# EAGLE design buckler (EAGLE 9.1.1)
AUTHOR: Branden Ghena; REV: C; TITLE: Berkeley Buckler

## Sheet 1 of 3: Headers
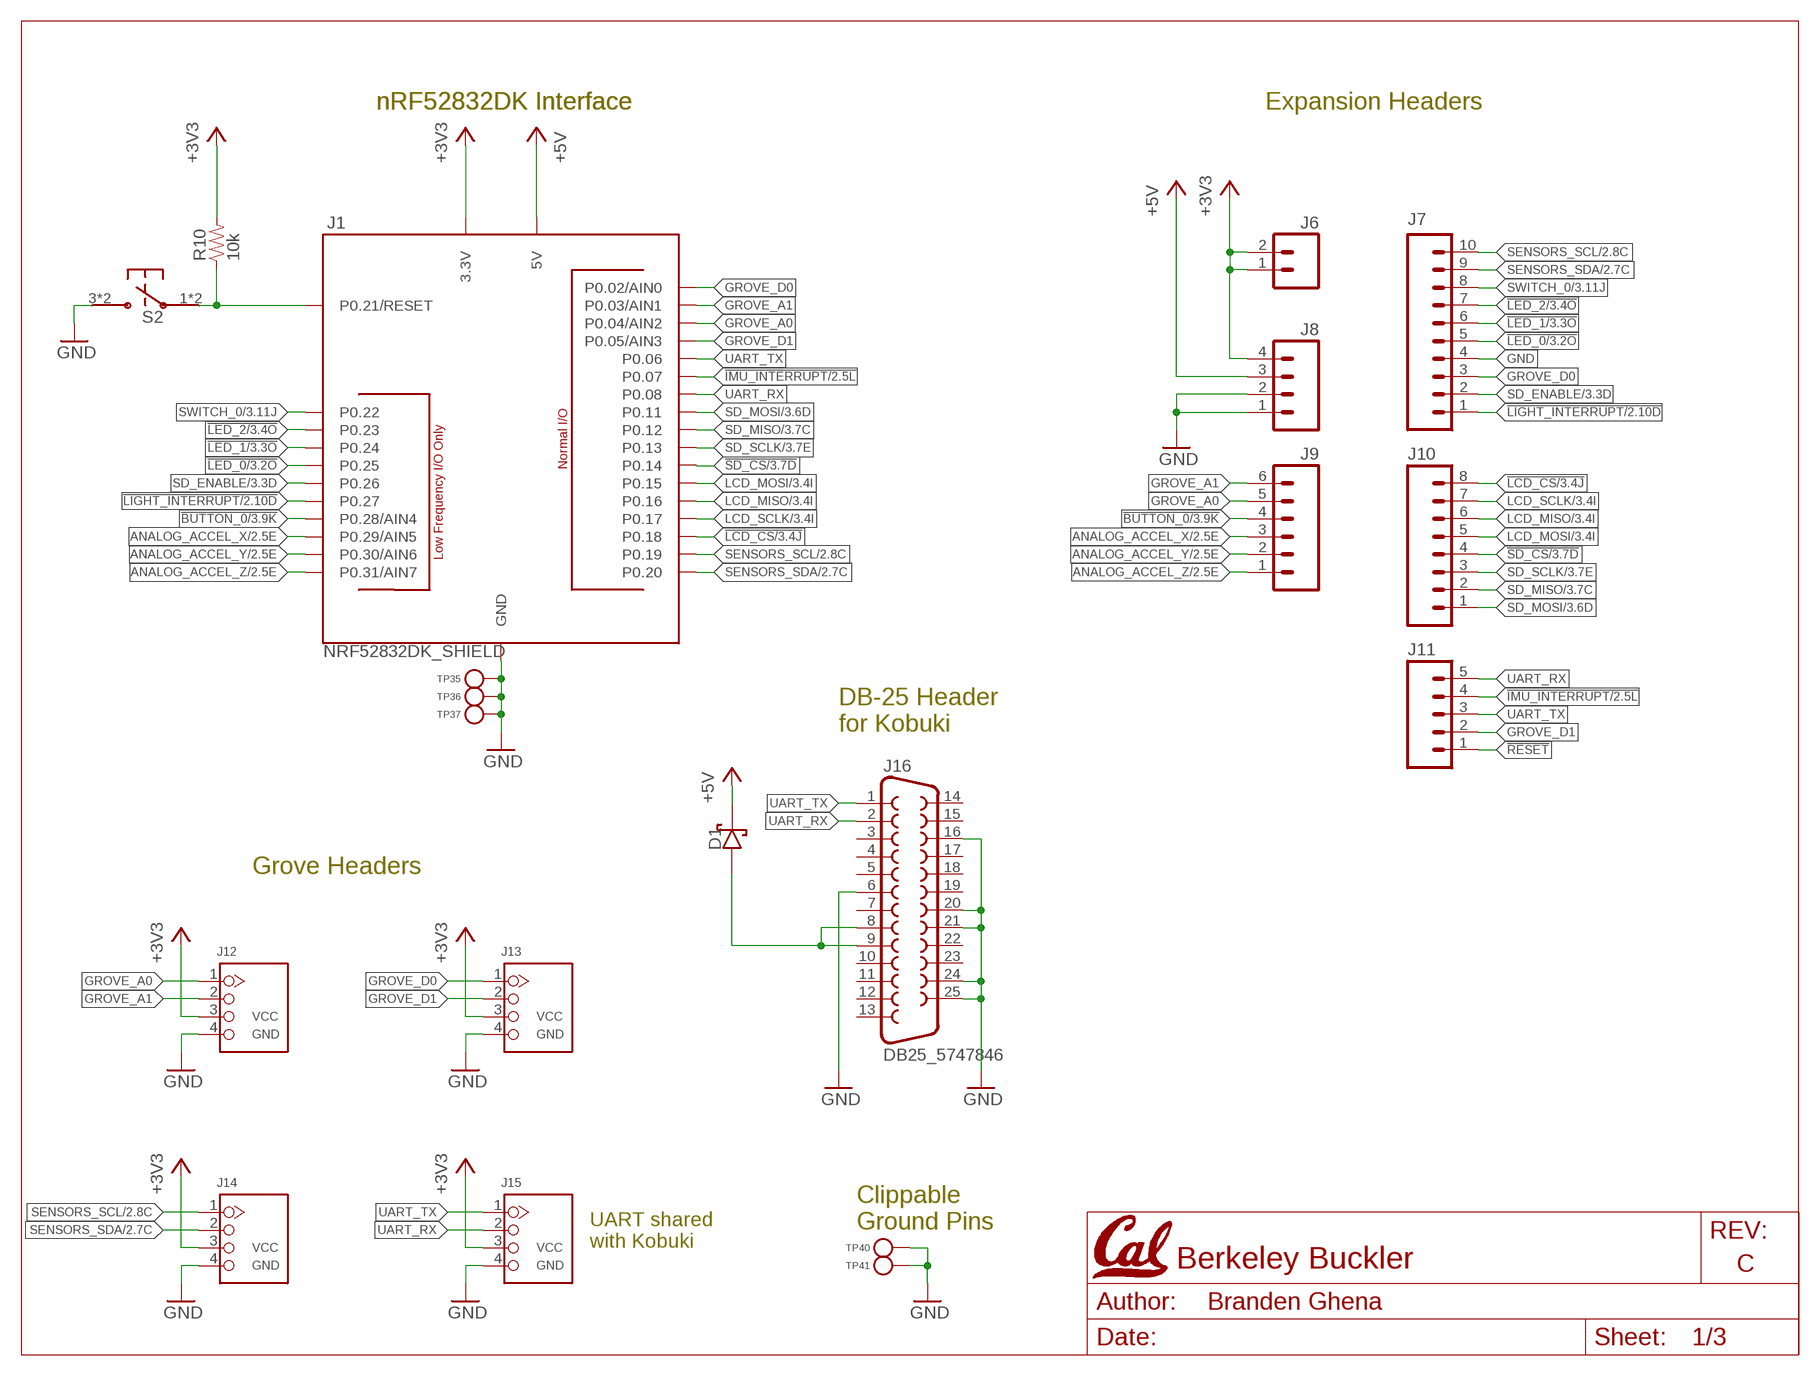
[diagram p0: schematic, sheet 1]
U$1 (LETTER_L_CAL): HEIGHT: 8.5in; WIDTH: 11in

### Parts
D1  DIODE_SCHOTTKYSOD323  [SOD323]
J1  NRF52832DK_SHIELD  [NRF52832DK_SHIELD]
J6  M02PTH  [1X02]
J7  M10"  [1X10]
J8  M04PTH  [1X04]
J9  M06SIP  [1X06]
J10  M081X08  [1X08]
J11  M05PTH  [1X05]
J12  GROVE-CONNECTOR-DIP(4P-2.0)  [HW4-2.0]
J13  GROVE-CONNECTOR-DIP(4P-2.0)  [HW4-2.0]
J14  GROVE-CONNECTOR-DIP(4P-2.0)  [HW4-2.0]
J15  GROVE-CONNECTOR-DIP(4P-2.0)  [HW4-2.0]
J16  DB25_5747846  [DB25_5747846]
R10  10k  RESISTOR0402_RES  [0402_RES]
S2  PTS645SM43SMTR92  [PTS645]
TP35  TEST_POINT_0.040IN  [TESTPOINT_0.040IN]
TP36  TEST_POINT_0.040IN  [TESTPOINT_0.040IN]
TP37  TEST_POINT_0.040IN  [TESTPOINT_0.040IN]
TP40  TEST_POINT_0.078IN  [TESTPOINT_0.078IN]
TP41  TEST_POINT_0.078IN  [TESTPOINT_0.078IN]

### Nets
5V_IN: D1.P$2(ANODE) J16.8 J16.9
!BUTTON_0: J1.P0.28(P0.28/AIN4) J9.4 ; also sheet 3
!IMU_INTERRUPT: J1.P0.07 J11.4 ; also sheet 2
!LCD_CS: J1.P0.18 J10.8 ; also sheet 3
!LED_0: J1.P0.25 J7.5 ; also sheet 3
!LED_1: J1.P0.24 J7.6 ; also sheet 3
!LED_2: J1.P0.23 J7.7 ; also sheet 3
!LIGHT_INTERRUPT: J1.P0.27 J7.1 ; also sheet 2
!RESET: J1.P0.21(P0.21/RESET) J11.1 R10.1 S2.1 S2.2
!SD_CS: J1.P0.14 J10.4 ; also sheet 3
+3V3: J1.3.3V@0(3.3V) J1.3.3V@1(3.3V) J1.3.3V@2(3.3V) J6.1 J6.2 J8.4 J12.3 J13.3 J14.3 J15.3 R10.2 ; also sheet 2,3
+5V: D1.P$1(CATHODE) J1.5V J8.3
ANALOG_ACCEL_X: J1.P0.29(P0.29/AIN5) J9.3 ; also sheet 2
ANALOG_ACCEL_Y: J1.P0.30(P0.30/AIN6) J9.2 ; also sheet 2
ANALOG_ACCEL_Z: J1.P0.31(P0.31/AIN7) J9.1 ; also sheet 2
GND: J1.GND@0(GND) J1.GND@1(GND) J1.GND@2(GND) J7.4 J8.1 J8.2 J12.4 J13.4 J14.4 J15.4 J16.6 J16.16 J16.20 J16.21 J16.24 J16.25 S2.3 S2.4 TP35.TESTPOINT TP36.TESTPOINT TP37.TESTPOINT TP40.1(TESTPOINT) TP41.1(TESTPOINT) ; also sheet 2,3
GROVE_A0: J1.P0.04(P0.04/AIN2) J9.5 J12.1
GROVE_A1: J1.P0.03(P0.03/AIN1) J9.6 J12.2
GROVE_D0: J1.P0.02(P0.02/AIN0) J7.3 J13.1
GROVE_D1: J1.P0.05(P0.05/AIN3) J11.2 J13.2
LCD_MISO: J1.P0.16 J10.6 ; also sheet 3
LCD_MOSI: J1.P0.15 J10.5 ; also sheet 3
LCD_SCLK: J1.P0.17 J10.7 ; also sheet 3
SD_ENABLE: J1.P0.26 J7.2 ; also sheet 3
SD_MISO: J1.P0.12 J10.2 ; also sheet 3
SD_MOSI: J1.P0.11 J10.1 ; also sheet 3
SD_SCLK: J1.P0.13 J10.3 ; also sheet 3
SENSORS_SCL: J1.P0.19 J7.10 J14.1 ; also sheet 2
SENSORS_SDA: J1.P0.20 J7.9 J14.2 ; also sheet 2
SWITCH_0: J1.P0.22 J7.8 ; also sheet 3
UART_RX: J1.P0.08 J11.5 J15.2 J16.2
UART_TX: J1.P0.06 J11.3 J15.1 J16.1
Unconnected: J16.3 J16.4 J16.5 J16.7 J16.10 J16.11 J16.12 J16.13 J16.14 J16.15 J16.17 J16.18 J16.19 J16.22 J16.23

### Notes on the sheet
- nRF52832DK Interface | nRF52832DK Interface | Expansion Headers
- DB-25 Header
  for Kobuki
- Grove Headers
- Clippable
  Ground Pins
- UART shared
  with Kobuki

## Sheet 2 of 3: Sensors
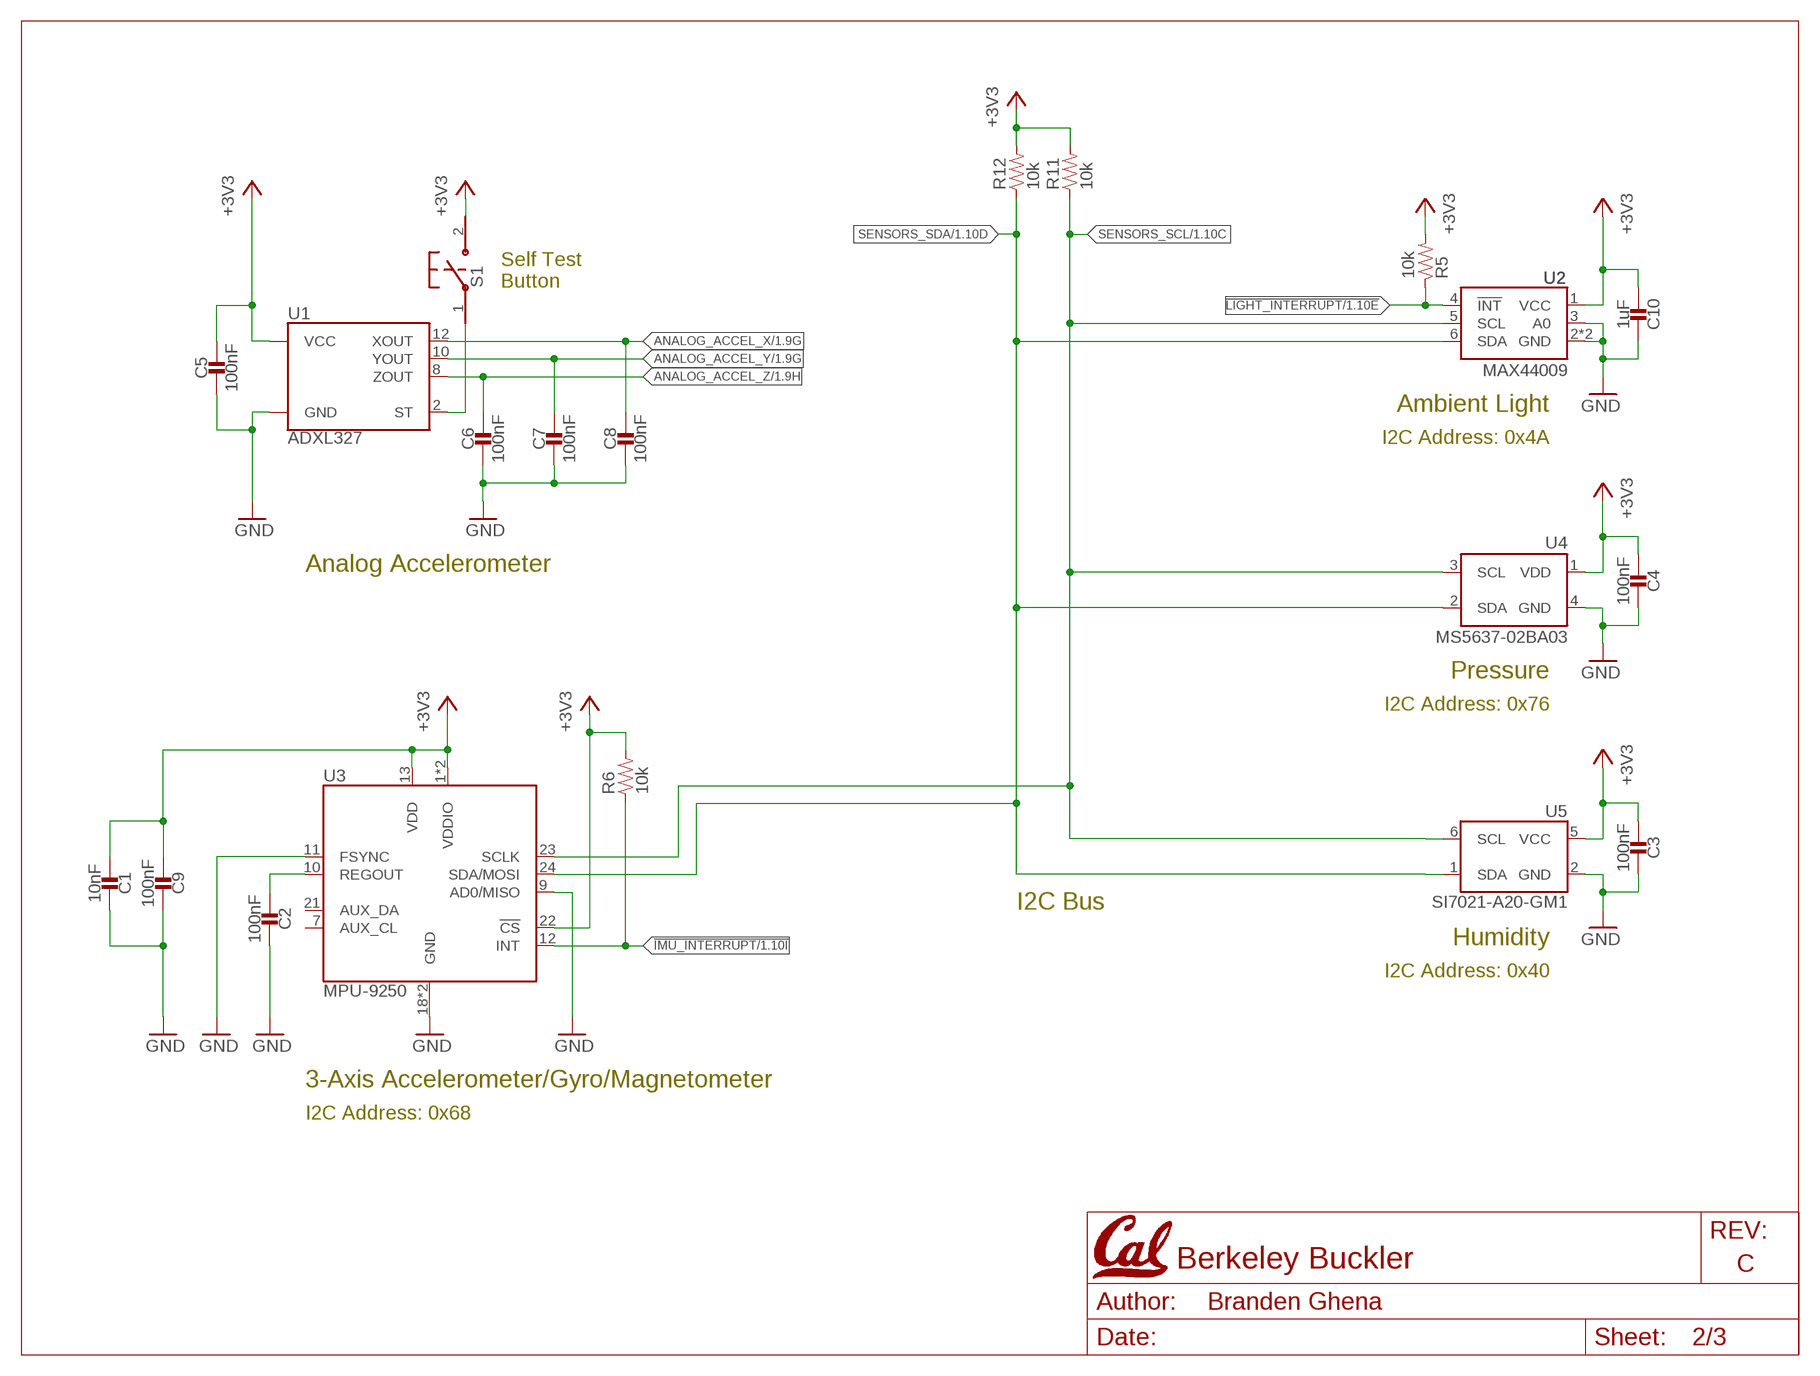
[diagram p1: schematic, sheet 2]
U$2 (LETTER_L_CAL): HEIGHT: 8.5in; WIDTH: 11in

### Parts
C1  10nF  CAPACITOR0402_CAP  [0402_CAP]
C2  100nF  CAPACITOR0402_CAP  [0402_CAP]
C3  100nF  CAPACITOR0402_CAP  [0402_CAP]
C4  100nF  CAPACITOR0402_CAP  [0402_CAP]
C5  100nF  CAPACITOR0402_CAP  [0402_CAP]
C6  100nF  CAPACITOR0402_CAP  [0402_CAP]
C7  100nF  CAPACITOR0402_CAP  [0402_CAP]
C8  100nF  CAPACITOR0402_CAP  [0402_CAP]
C9  100nF  CAPACITOR0402_CAP  [0402_CAP]
C10  1uF  CAPACITOR0402_CAP  [0402_CAP]
R5  10k  RESISTOR0402_RES  [0402_RES]
R6  10k  RESISTOR0402_RES  [0402_RES]
R11  10k  RESISTOR0402_RES  [0402_RES]
R12  10k  RESISTOR0402_RES  [0402_RES]
S1  B3U-1000P  [B3U-1000P]
U1  ADXL327  [LFCSP-16]
U2  MAX44009  [UDFN-6-EXPOSED]
U3  MPU-9250  [QFN-24/3MM]
U4  MS5637-02BA03  [4-SMD]
U5  SI7021-A20-GM1  [DFN-6/3MM]

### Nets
!IMU_INTERRUPT: R6.1 U3.12(INT) ; also sheet 1
!LIGHT_INTERRUPT: R5.1 U2.4(!INT) ; also sheet 1
+3V3: C1.1 C3.1 C4.1 C5.1 C9.1 C10.1 R5.2 R6.2 R11.2 R12.2 S1.2 U1.14(VCC) U1.15(VCC) U2.1(VCC) U3.1(VDDIO) U3.8(VDDIO) U3.13(VDD) U3.22(!CS) U4.1(VDD) U5.5(VCC) ; also sheet 1,3
ANALOG_ACCEL_X: C8.1 U1.12(XOUT) ; also sheet 1
ANALOG_ACCEL_Y: C7.1 U1.10(YOUT) ; also sheet 1
ANALOG_ACCEL_Z: C6.1 U1.8(ZOUT) ; also sheet 1
GND: C1.2 C2.2 C3.2 C4.2 C5.2 C6.2 C7.2 C8.2 C9.2 C10.2 U1.3(GND) U1.5(GND) U1.6(GND) U1.7(GND) U2.2(GND) U2.3(A0) U2.EP(GND) U3.9(AD0/MISO) U3.11(FSYNC) U3.18(GND) U3.20(GND) U4.4(GND) U5.2(GND) ; also sheet 1,3
N$7: S1.1 U1.2(ST)
N$19: C2.1 U3.10(REGOUT)
SENSORS_SCL: R11.1 U2.5(SCL) U3.23(SCLK) U4.3(SCL) U5.6(SCL) ; also sheet 1
SENSORS_SDA: R12.1 U2.6(SDA) U3.24(SDA/MOSI) U4.2(SDA) U5.1(SDA) ; also sheet 1
Unconnected: U3.7(AUX_CL) U3.21(AUX_DA)

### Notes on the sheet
- Self Test
  Button
- Ambient Light
- I2C Address: 0x4A
- Analog Accelerometer
- Pressure
- I2C Address: 0x76
- I2C Bus
- Humidity
- I2C Address: 0x40
- 3-Axis Accelerometer/Gyro/Magnetometer
- I2C Address: 0x68

## Sheet 3 of 3: Other Peripherals
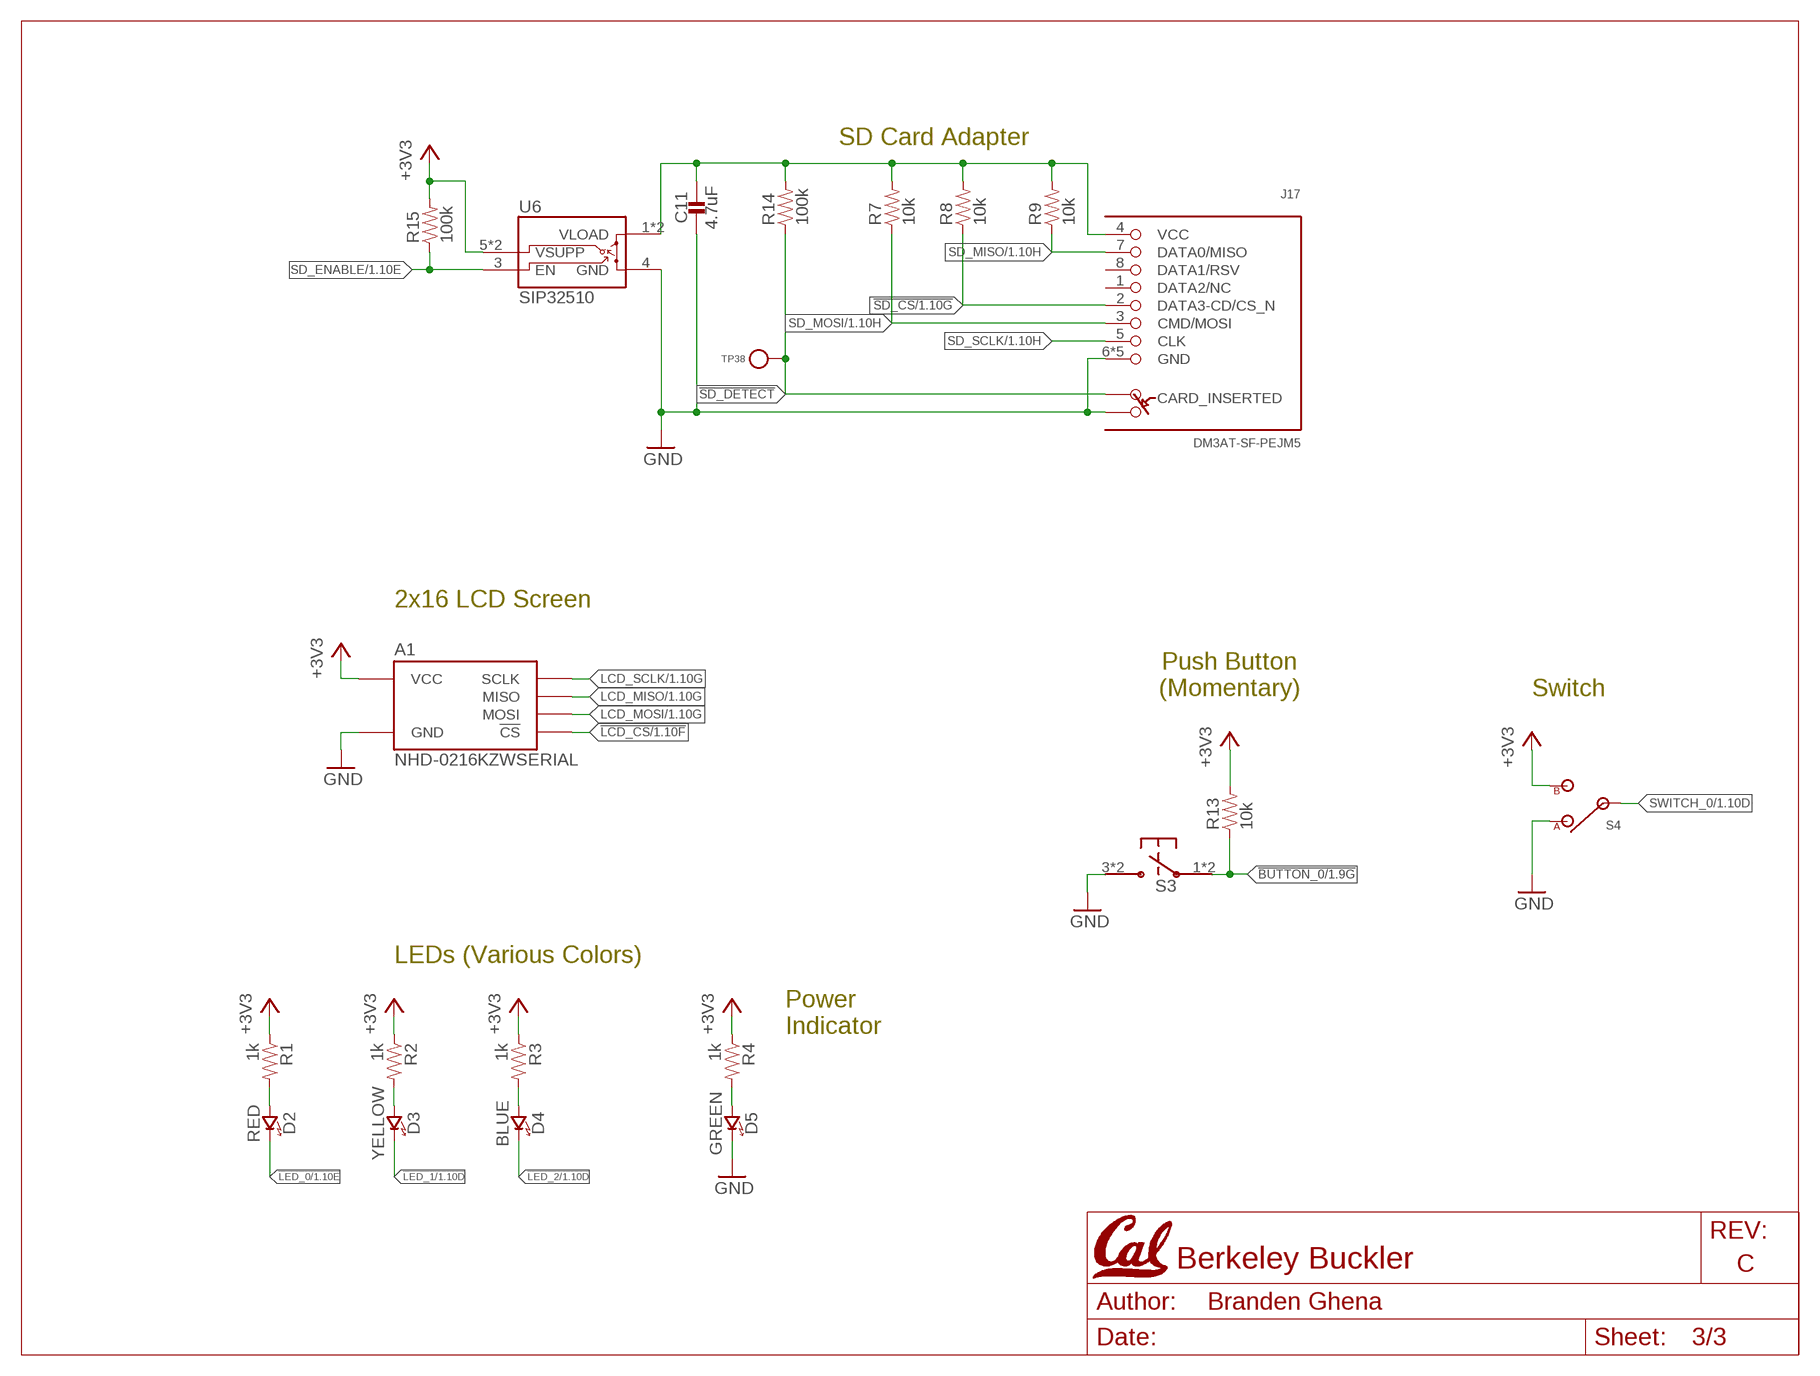
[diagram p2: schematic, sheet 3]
U$3 (LETTER_L_CAL): HEIGHT: 8.5in; WIDTH: 11in

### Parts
A1  NHD-0216KZWSERIAL  [NHD-0216KZW]
C11  4.7uF  CAPACITOR0402_CAP  [0402_CAP]
D2  RED  LED0603  [LED-0603]
D3  YELLOW  LED0603  [LED-0603]
D4  BLUE  LED0603  [LED-0603]
D5  GREEN  LED0603  [LED-0603]
J17  DM3AT-SF-PEJM5  [DM3AT-SF-PEJM5]
R1  1k  RESISTOR0402_RES  [0402_RES]
R2  1k  RESISTOR0402_RES  [0402_RES]
R3  1k  RESISTOR0402_RES  [0402_RES]
R4  1k  RESISTOR0402_RES  [0402_RES]
R7  10k  RESISTOR0402_RES  [0402_RES]
R8  10k  RESISTOR0402_RES  [0402_RES]
R9  10k  RESISTOR0402_RES  [0402_RES]
R13  10k  RESISTOR0402_RES  [0402_RES]
R14  100k  RESISTOR0402_RES  [0402_RES]
R15  100k  RESISTOR0402_RES  [0402_RES]
S3  PTS645SM43SMTR92  [PTS645]
S4  TE_SSA12/SPDT  [TE_SSA12/SPDT]
TP38  TEST_POINT_0.040IN  [TESTPOINT_0.040IN]
U6  SIP32510  [TSOT23-6]

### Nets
!BUTTON_0: R13.1 S3.1 S3.2 ; also sheet 1
!LCD_CS: A1.16(!CS) ; also sheet 1
!LED_0: D2.C(CATHODE) ; also sheet 1
!LED_1: D3.C(CATHODE) ; also sheet 1
!LED_2: D4.C(CATHODE) ; also sheet 1
!SD_CS: J17.2(DATA3-CD/CS_N) R8.1 ; also sheet 1
!SD_DETECT: J17.A R14.1 TP38.TESTPOINT
+3V3: A1.2(VCC) R1.1 R2.1 R3.1 R4.1 R13.2 R15.2 S4.2(B) U6.5(VSUPP) U6.6(VSUPP) ; also sheet 1,2
GND: A1.1(GND) C11.2 D5.C(CATHODE) J17.6(GND) J17.B J17.MOUNT0(GND) J17.MOUNT1(GND) J17.MOUNT2(GND) J17.MOUNT3(GND) S3.3 S3.4 S4.1(A) U6.4(GND) ; also sheet 1,2
LCD_MISO: A1.13(MISO) ; also sheet 1
LCD_MOSI: A1.14(MOSI) ; also sheet 1
LCD_SCLK: A1.12(SCLK) ; also sheet 1
N$3: D5.A(ANODE) R4.2
N$4: D4.A(ANODE) R3.2
N$5: D3.A(ANODE) R2.2
N$18: C11.1 J17.4(VCC) R7.2 R8.2 R9.2 R14.2 U6.1(VLOAD) U6.2(VLOAD)
N$25: D2.A(ANODE) R1.2
SD_ENABLE: R15.1 U6.3(EN) ; also sheet 1
SD_MISO: J17.7(DATA0/MISO) R9.1 ; also sheet 1
SD_MOSI: J17.3(CMD/MOSI) R7.1 ; also sheet 1
SD_SCLK: J17.5(CLK) ; also sheet 1
SWITCH_0: S4.IN ; also sheet 1
Unconnected: J17.1(DATA2/NC) J17.8(DATA1/RSV)

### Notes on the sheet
- SD Card Adapter
- 2x16 LCD Screen
- Push Button
  (Momentary)
- Switch
- LEDs (Various Colors)
- Power
  Indicator

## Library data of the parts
A1 = headers:NHD-0216KZW; DIGIKEY: NHD-0216KZW-AG5-ND,952-3305-ND; DIGIKEY1: NHD-0216KZW-AG5-ND; DIGIKEY2: 952-3305-ND; DIGIKEY3: 952-1862-ND
C1 = passives:CAPACITOR: SMD Capacitor; DESCRIPTION: CAP CER 10000PF 25V X7R 0402; DIGIKEY: 399-1279-1-ND; MANUFACTURER: KEMET; MPN: C0402C103J3RACTU
C2-C9 = passives:CAPACITOR: SMD Capacitor; DESCRIPTION: CAP CER 0.1UF 16V X7R 0402; DIGIKEY: 490-4759-1-ND; MANUFACTURER: Murata; MPN: GCM155R71C104KA55D
C10 = passives:CAPACITOR: SMD Capacitor; DESCRIPTION: CAP CER 1UF 10V X6S 0402; DIGIKEY: 1276-6805-1-ND; MANUFACTURER: Samsung Electro-Mechanics; MPN: CL05X105KP5NNNC
C11 = passives:CAPACITOR: SMD Capacitor; DESCRIPTION: CAP CER 4.7UF 10V X5R 0402; DIGIKEY: 1276-1480-1-ND; MANUFACTURER: Samsung Electro-Mechanics; MPN: CL05A475KP5NRNC
D1 = passives:DIODE_SCHOTTKY; DESCRIPTION: DIODE SCHOTTKY 30V 500MA SOD323; DIGIKEY: B0530WS-FDICT-ND; MANUFACTURER: Diodes Incorporated; MPN: B0530WS-7-F
D2 = leds:LED: LED; DESCRIPTION: LED RED CLEAR CHIP SMD; DIGIKEY: 160-1436-1-ND; MANUFACTURER: Lite-On Inc.; MPN: LTST-C190KRKT
D3 = leds:LED: LED; DESCRIPTION: LED YELLOW CLEAR CHIP SMD; DIGIKEY: 160-1437-1-ND; MANUFACTURER: Lite-On Inc.; MPN: LTST-C190KSKT
D4 = leds:LED: LED; DESCRIPTION: LED BLUE CLEAR SMD; DIGIKEY: 160-1837-1-ND; MANUFACTURER: Lite-On Inc.; MPN: LTST-C194TBKT
D5 = leds:LED: LED; DESCRIPTION: LED GREEN CLEAR CHIP SMD; DIGIKEY: 160-1435-1-ND; MANUFACTURER: Lite-On Inc.; MPN: LTST-C190KGKT
J1 = headers:NRF52832DK_SHIELD: Shield for the PCA10040 nRF52832 Development Kit; DIGIKEY1: S1011EC-10-ND; DIGIKEY2: S1011EC-08-ND; DIGIKEY3: S1011EC-08-ND; DIGIKEY4: S1011EC-06-ND; DIGIKEY5: S1011EC-09-ND
J6 = SparkFun-Connectors:M02: Header 2; DIGIKEY: S1011EC-02-ND
J7 = SparkFun-Connectors:M10: Header 10 Standard 10-pin 0.1" header. Use with straight break away headers (SKU : PRT-00116), right angle break away headers (PRT-00553), swiss pins (PRT-00743), machine pins (PRT-00117), and female headers (PRT-00115).; DIGIKEY: S1011EC-10-ND
J8 = SparkFun-Connectors:M04: Header 4 Standard 4-pin 0.1" header. Use with straight break away headers (SKU : PRT-00116), right angle break away headers (PRT-00553), swiss pins (PRT-00743), machine pins (PRT-00117), and female headers (PRT-00115). Molex polarized connector foot print use with SKU : PRT-08231 with associated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; DIGIKEY: S1011EC-04-ND
J9 = SparkFun-Connectors:M06: Header 6 Standard 6-pin 0.1" header. Use with straight break away headers (SKU : PRT-00116), right angle break away headers (PRT-00553), swiss pins (PRT-00743), machine pins (PRT-00117), and female headers (PRT-00115). Molex polarized connector foot print use with SKU : PRT-08094 with associated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; DIGIKEY: S1011EC-06-ND
J10 = SparkFun-Connectors:M08: Header 8 Standard 8-pin 0.1" header. Use with straight break away headers (SKU : PRT-00116), right angle break away headers (PRT-00553), swiss pins (PRT-00743), machine pins (PRT-00117), and female headers (PRT-00115).; DIGIKEY: S1011EC-08-ND
J11 = SparkFun-Connectors:M05: Header 5 Standard 5-pin 0.1" header. Use with straight break away headers (SKU : PRT-00116), right angle break away headers (PRT-00553), swiss pins (PRT-00743), machine pins (PRT-00117), and female headers (PRT-00115). Molex polarized connector foot print use with SKU : PRT-08230 with associated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; DIGIKEY: S1011EC-05-ND
J12-J15 = headers:GROVE-CONNECTOR-DIP(4P-2.0): 320110033; DESCRIPTION: Grove - Universal 4 pin connector; MANUFACTURER: Seeed Studio; MOUSER: 713-110990030; MPN: 110990030; VALUE: 4P-2.0
J16 = headers:DB25_5747846; DESCRIPTION: CONN D-SUB RCPT 25POS R/A SOLDER; DIGIKEY: A32126-ND; MANUFACTURER: TE Connectivity AMP Connectors; MPN: 5747846-4
J17 = connector:DM3AT-SF-PEJM5: CONN MICRO SD R/A PUSH-PUSH SMD; DESCRIPTION: CONN MICRO SD CARD PUSH-PUSH R/A; DIGIKEY: HR1964CT-ND; MANUFACTURER: Hirose Electric Co Ltd; MPN: DM3AT-SF-PEJM5
R1-R4 = passives:RESISTOR: Resistor; DESCRIPTION: RES SMD 1K OHM 1% 1/16W 0402; DIGIKEY: RMCF0402FT1K00CT-ND; MANUFACTURER: Stackpole Electronics; MPN: RMCF0402FT1K00
R5-R13 = passives:RESISTOR: Resistor; DESCRIPTION: RES SMD 10K OHM 1% 1/16W 0402; DIGIKEY: 1276-3431-1-ND; MANUFACTURER: Samsung Electro-Mechanics; MPN: RC1005F103CS
R14 R15 = passives:RESISTOR: Resistor; DESCRIPTION: RES SMD 100K OHM 1% 1/5W 0402; DIGIKEY: 541-100KYCT-ND; MANUFACTURER: Vishay Dale; MPN: CRCW0402100KFKEDHP
S1 = switches:B3U: Switch; DESCRIPTION: SWITCH TACTILE SPST-NO 0.05A 12V; DIGIKEY: SW1020CT-ND; MANUFACTURER: Omron; MPN: B3U-1000P
S2 S3 = switches:PTS645SM43SMTR92: Tactile Switch SPST-NO Top Actuated Surface Mount; DESCRIPTION: SWITCH TACTILE SPST-NO 0.05A 12V; DIGIKEY: CKN9112CT-ND; MANUFACTURER: C&K; MPN: PTS645SM43SMTR92 LFS
S4 = switches:TE_SSA12/SPDT: SWITCH SLIDE SPDT 2POS SSA SER; DESCRIPTION: SWITCH SLIDE SPDT 100MA 30V; DIGIKEY: 450-1602-ND; MANUFACTURER: TE Connectivity ALCOSWITCH Switches; MPN: SSA12
TP35-TP38 = headers:TEST_POINT_0.040IN: 0.040in Test Point; DIGIKEY: 5001K-ND
TP40 TP41 = headers:TEST_POINT_0.078IN; DESCRIPTION: TERM TURRET SINGLE L=4.75MM TIN; DIGIKEY: 36-1520-2-ND; MANUFACTURER: Keystone Electronics; MPN: 1520-2
U1 = chips:ADXL327: ADXL327 3-Axis Analog Accelerometer; DESCRIPTION: ACCELEROMETER 2G ANALOG 16LFCSP; DIGIKEY: ADXL327BCPZ-ND; MANUFACTURER: Analog Devices Inc.; MPN: ADXL327BCPZ
U2 = chips:MAX44009: low power ambient light sensor; DESCRIPTION: SENSOR AMBIENT LIGHT 6UTDFN; DIGIKEY: MAX44009EDT+TCT-ND; MANUFACTURER: Maxim Integrated; MPN: MAX44009EDT+T
U3 = chips:MPU-9250: GYRO/ACCEL/COMPASS/9-AXIS; DESCRIPTION: IMU ACCEL/GYRO/MAG I2C/SPI 24QFN; DIGIKEY: 1428-1019-1-ND; MANUFACTURER: TDK InvenSense; MPN: MPU-9250
U4 = chips:MS5637-02BA03: low power pressure sensor; DESCRIPTION: SENSOR 17.4PSIA I2C 24B 4-QFN; DIGIKEY: 223-1199-1-ND; MANUFACTURER: TE CONNECTIVITY; MPN: MS563702BA03-50
U5 = chips:SI7021: IC TEMP SENSOR RH 2% DFN; DESCRIPTION: SENS HUMI/TEMP 3.6V I2C 3% 6DFN; DIGIKEY: 336-3141-ND; MANUFACTURER: Silicon Labs; MOUSER: 634-SI7021-A20-GM1; MPN: SI7021-A20-GM1
U6 = chips:SIP32510: Load switch, slew rate controlled. By Vishay; DESCRIPTION: IC LOAD SWITCH SOT23-6; DIGIKEY: SIP32510DT-T1-GE3CT-ND; MANUFACTURER: Vishay; MPN: SIP32510DT-T1-GE3

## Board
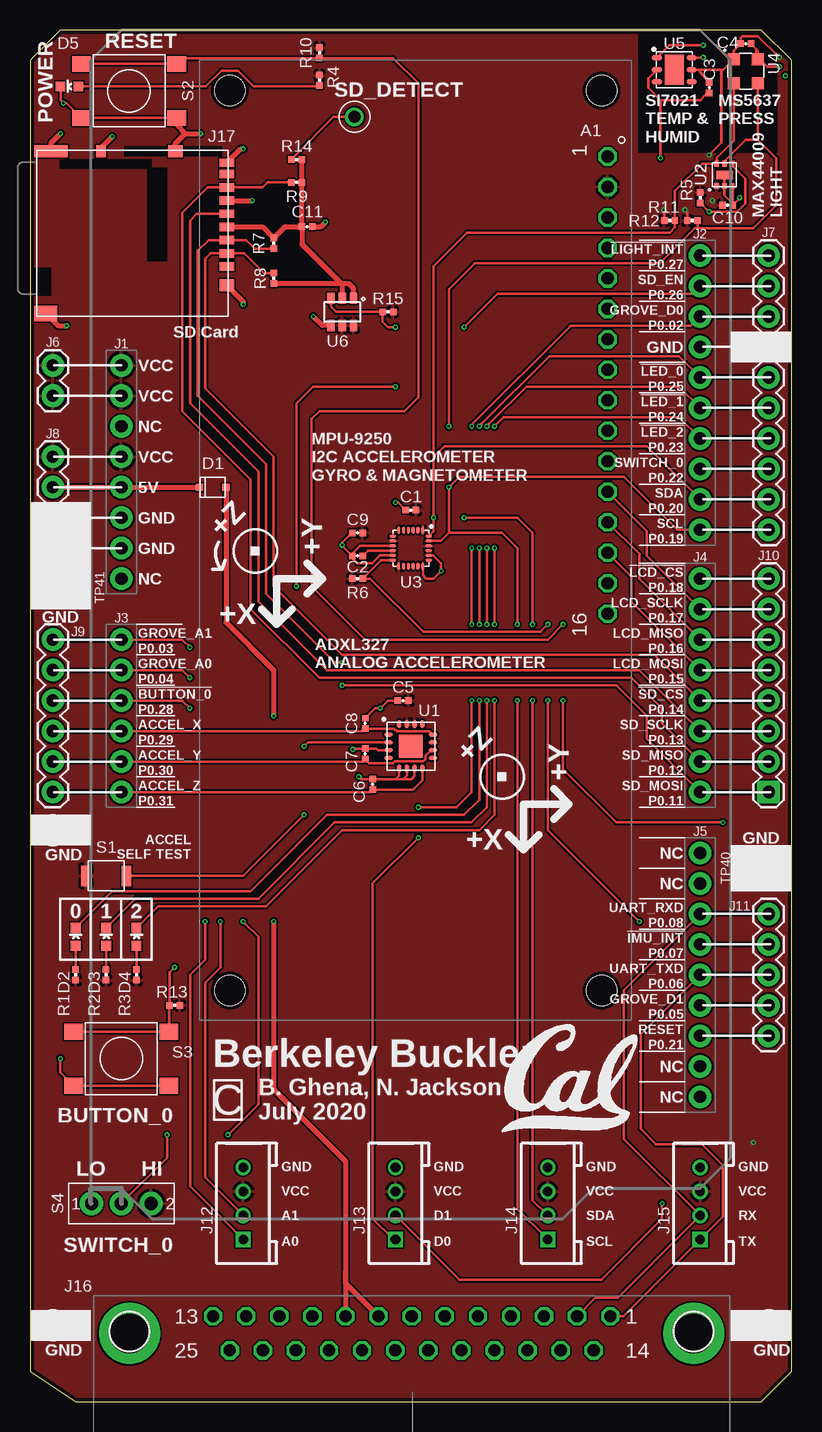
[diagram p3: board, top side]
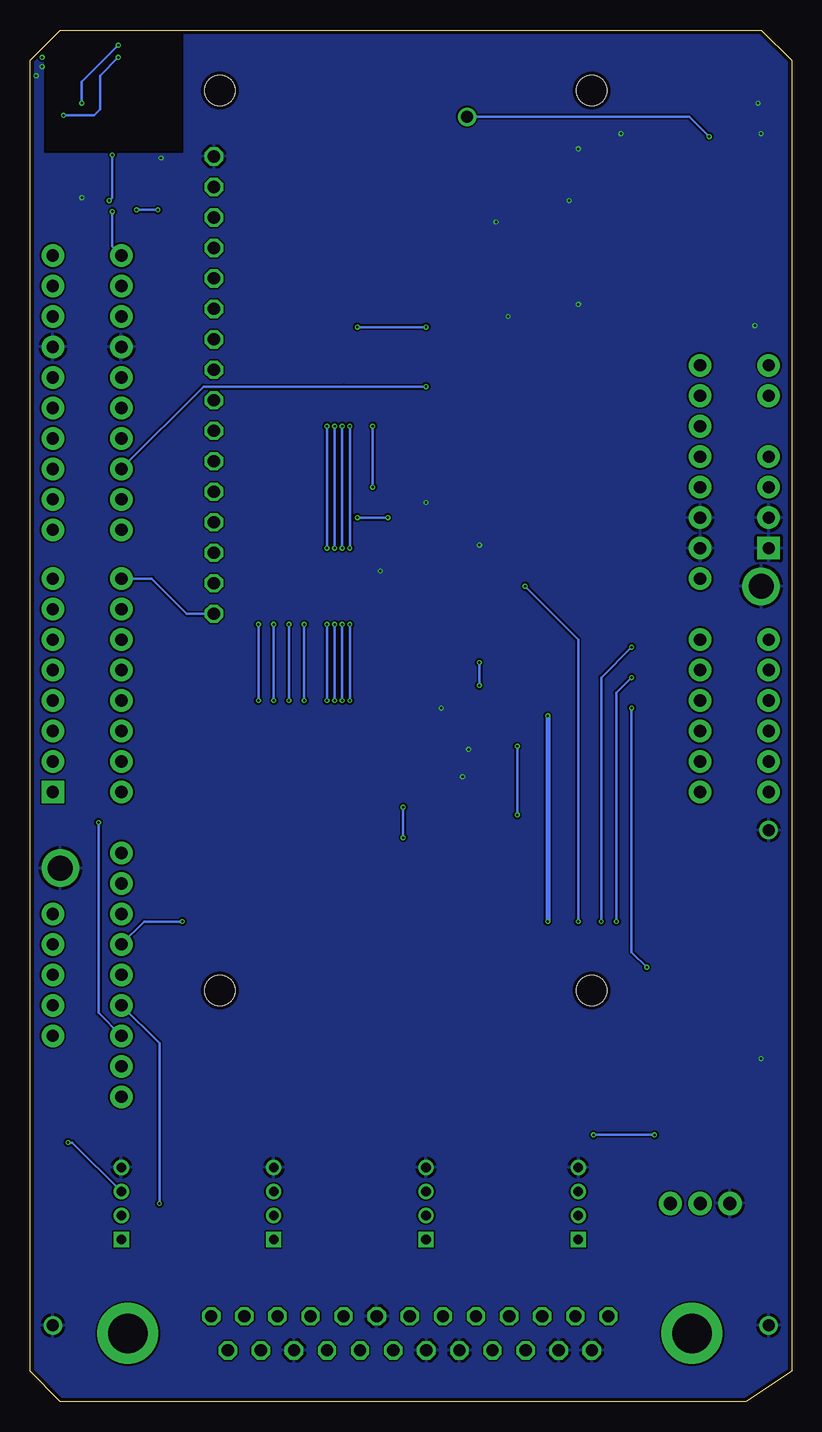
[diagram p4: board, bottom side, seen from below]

Size 63.5 x 114.3 mm. Coordinates in mm from the lower left corner, seen from the top.
Outline: 60.96,114.3 2.54,114.3 0,111.76 0,2.54 3.81,0 60.96,0 63.5,2.54 63.5,111.76 60.96,114.3
Copper layers (1*16): Top 0.0178mm / dielectric 59mil / Bottom 0.0178mm
Design rules "quickturn_co_kr_1oz": minimum track width 4mil, minimum drill 0.200659375mm, track to track 6mil, track to pad 6mil, pad to pad 6mil, via to via 6mil, smd to smd 6mil, copper to edge 12mil, drill to drill 12mil, minimum pad ring 8mil, minimum via ring 4mil, stop-mask expansion 3mil, vias tented up to drill 50mil, thermal gap 10mil

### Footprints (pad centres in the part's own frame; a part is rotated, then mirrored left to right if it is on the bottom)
NHD-0216KZW = drill 1.016 octagon: 1 8,-2; 2 10.54,-2; 3 13.08,-2; 4 15.62,-2; 5 18.16,-2; 6 20.7,-2; 7 23.24,-2; 8 25.78,-2; 9 28.32,-2; 10 30.86,-2; 11 33.4,-2; 12 35.94,-2; 13 38.48,-2; 14 41.02,-2; 15 43.56,-2; 16 46.1,-2 | hole 2.5: 2.5,-2.5; 2.5,-33.5; 77.5,-33.5; 77.5,-2.5
0402_CAP = smd 0.536 x 0.546: 1 -0.433,0; 2 0.433,0
SOD323 = smd 0.6 x 0.6: P$1 -1.1,0; P$2 1.1,0
LED-0603 = smd 0.8 x 0.8: A 0,-0.75; C 0,0.75
NRF52832DK_SHIELD = drill 1.016 pad 1.88: 3.3V@0 0,-7.62; 3.3V@1 0,-2.54; 3.3V@2 0,0; 5V 0,-10.16; !RESET 0,-5.08; GND@0 0,-12.7; GND@1 0,-15.24; GND@2 48.26,1.524; NC@0 0,-17.78; NC@1 48.26,-58.42; NC@2 48.26,-60.96; P0.02 48.26,4.064; P0.03 0,-22.86; P0.04 0,-25.4; P0.05 48.26,-53.34; P0.06 48.26,-50.8; P0.07 48.26,-48.26; P0.08 48.26,-45.72; P0.09 48.26,-43.18; P0.10 48.26,-40.64; P0.11 48.26,-35.56; P0.12 48.26,-33.02; P0.13 48.26,-30.48; P0.14 48.26,-27.94; P0.15 48.26,-25.4; P0.16 48.26,-22.86; P0.17 48.26,-20.32; P0.18 48.26,-17.78; P0.19 48.26,-13.716; P0.20 48.26,-11.176; P0.21 48.26,-55.88; P0.22 48.26,-8.636; P0.23 48.26,-6.096; P0.24 48.26,-3.556; P0.25 48.26,-1.016; P0.26 48.26,6.604; P0.27 48.26,9.144; P0.28 0,-27.94; P0.29 0,-30.48; P0.30 0,-33.02; P0.31 0,-35.56
1X02 = drill 1.016 pad 1.88: 1 0,0; 2 2.54,0
1X10 = drill 1.016 pad 1.88: 1 0,0; 2 2.54,0; 3 5.08,0; 4 7.62,0; 5 10.16,0; 6 12.7,0; 7 15.24,0; 8 17.78,0; 9 20.32,0; 10 22.86,0
1X04 = drill 1.016 pad 1.88 square: 1 0,0 | drill 1.016 pad 1.88: 2 2.54,0; 3 5.08,0; 4 7.62,0
1X06 = drill 1.016 pad 1.88: 1 0,0; 2 2.54,0; 3 5.08,0; 4 7.62,0; 5 10.16,0; 6 12.7,0
1X08 = drill 1.016 pad 1.88 square: 1 0,0 | drill 1.016 pad 1.88: 2 2.54,0; 3 5.08,0; 4 7.62,0; 5 10.16,0; 6 12.7,0; 7 15.24,0; 8 17.78,0
1X05 = drill 1.016 pad 1.88: 1 0,0; 2 2.54,0; 3 5.08,0; 4 7.62,0; 5 10.16,0
HW4-2.0 = drill 0.8 pad 1.27 square: 1 -3,0 | drill 0.8 pad 1.27: 2 -1,0; 3 1,0; 4 3,0
DB25_5747846 = drill 1.016 octagon: 1 0,0; 2 2.76,0; 3 5.52,0; 4 8.28,0; 5 11.041,0; 6 13.801,0; 7 16.561,0; 8 19.321,0; 9 22.081,0; 10 24.841,0; 11 27.601,0; 12 30.362,0; 13 33.122,0; 14 1.379,2.845; 15 4.139,2.845; 16 6.898,2.845; 17 9.657,2.845; 18 12.417,2.845; 19 15.176,2.845; 20 17.935,2.845; 21 20.695,2.845; 22 23.454,2.845; 23 26.213,2.845; 24 28.973,2.845; 25 31.732,2.845 | drill 3.302 pad 5.08: G1 -6.96,1.422; G2 40.081,1.422
DM3AT-SF-PEJM5 = smd 0.7 x 1.2: 1 3.2,-0.1; 2 2.1,-0.1; 3 1,-0.1; 4 -0.1,-0.1; 5 -1.2,-0.1; 6 -2.3,-0.1; 7 -3.4,-0.1; 8 -4.5,-0.1; B -5.45,-0.1 | smd 1 x 0.8: A -6.4,-10.6 | smd 1 x 1.2: MOUNT0 4.75,-0.1; MOUNT1 -6.4,-4.4 | smd 1 x 2.8: MOUNT2 -6.4,-14.75 | smd 1.3 x 1.9: MOUNT3 7.1,-15.2
0402_RES = smd 0.536 x 0.546: 1 -0.433,0; 2 0.433,0
B3U-1000P = smd 0.8 x 1.7: 1 -1.7,0; 2 1.7,0
PTS645 = smd 1.55 x 1.3: 1 -3.975,2.25; 2 3.975,2.25; 3 3.975,-2.25; 4 -3.975,-2.25
TE_SSA12/SPDT = drill 1.092 pad 1.93: 1 -2.489,0; 2 2.489,0; IN 0,0
TESTPOINT_0.040IN = drill 1.016: TESTPOINT 0,0
TESTPOINT_0.078IN = drill 2.083: 1 0,0
LFCSP-16 = smd 0.7 x 0.35: 1 -1.85,0.975; 2 -1.85,0.325; 3 -1.85,-0.325; 4 -1.85,-0.975; 9 1.85,-0.975; 10 1.85,-0.325; 11 1.85,0.325; 12 1.85,0.975 | smd 0.35 x 0.7: 5 -0.975,-1.85; 6 -0.325,-1.85; 7 0.325,-1.85; 8 0.975,-1.85; 13 0.975,1.85; 14 0.325,1.85; 15 -0.325,1.85; 16 -0.975,1.85 | smd 1.95 x 1.95: PAD 0,0
UDFN-6-EXPOSED = smd 0.48 x 0.36: 1 -0.925,0.65; 2 -0.925,0; 3 -0.925,-0.65; 4 0.925,-0.65; 5 0.925,0; 6 0.925,0.65 | smd 0.71 x 1.4: EP 0,0
QFN-24/3MM = smd 0.6 x 0.23: 1 -1.5,1; 2 -1.5,0.6; 3 -1.5,0.2; 4 -1.5,-0.2; 5 -1.5,-0.6; 6 -1.5,-1; 13 1.5,-1; 14 1.5,-0.6; 15 1.5,-0.2; 16 1.5,0.2; 17 1.5,0.6; 18 1.5,1 | smd 0.23 x 0.6: 7 -1,-1.5; 8 -0.6,-1.5; 9 -0.2,-1.5; 10 0.2,-1.5; 11 0.6,-1.5; 12 1,-1.5; 19 1,1.5; 20 0.6,1.5; 21 0.2,1.5; 22 -0.2,1.5; 23 -0.6,1.5; 24 -1,1.5
4-SMD = smd 1 x 1: 1 -1,1; 2 -1,-1; 3 1,-1; 4 1,1
DFN-6/3MM = smd 0.85 x 0.45: 1 -1.45,1; 2 -1.45,0; 3 -1.45,-1; 4 1.45,-1; 5 1.45,0; 6 1.45,1 | smd 1.6 x 2.5: P$1 0,0
TSOT23-6 = smd 0.6 x 0.927: 1 -0.95,-1.126; 2 0,-1.126; 3 0.95,-1.126; 4 0.95,1.126; 5 0,1.126; 6 -0.95,1.126

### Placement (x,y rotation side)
A1  50.16,111.76 270 top
C1  31.75,74.29 180 top
C2  27.3,70.48 180 top
C3  56.64,109.47 270 top
C4  59.69,113.16 0 top
C5  31.11,58.42 180 top
C6  28.57,51.44 90 top
C7  27.94,53.98 90 top
C8  27.94,56.52 90 top
C9  27.3,72.39 180 top
C10  58.17,99.69 0 top
C11  23.11,97.92 0 top
D1  15.24,76.2 0 top
D2  3.81,38.73 0 top
D3  6.35,38.73 0 top
D4  8.89,38.73 0 top
D5  3.3,109.6 90 top
J1  7.62,86.36 0 top
J6  1.91,83.82 90 top
J7  61.59,95.5 270 top
J8  1.91,71.12 90 top
J9  1.91,50.8 90 top
J10  61.59,50.8 90 top
J11  61.59,30.48 90 top
J12  17.78,16.51 90 top
J13  30.48,16.51 90 top
J14  43.18,16.51 90 top
J15  55.88,16.51 90 top
J16  48.39,7.11 180 top
J17  16.51,97.79 270 top
R1  3.81,35.56 90 top
R2  6.35,35.56 90 top
R3  8.89,35.56 90 top
R4  24.13,110.11 270 top
R5  55.88,100.33 90 top
R6  27.3,68.58 180 top
R7  20.32,96.52 90 top
R8  20.32,93.6 270 top
R9  22.23,101.6 0 top
R10  24.13,112.39 90 top
R11  55.24,98.42 180 top
R12  53.34,98.42 180 top
R13  12.06,33.02 0 top
R14  22.23,103.5 0 top
R15  29.84,90.8 0 top
S1  6.35,43.82 180 top
S2  8.26,109.22 0 top
S3  7.62,28.58 0 top
S4  7.62,16.51 0 top
TP35  61.59,6.35 0 top
TP36  1.91,6.35 0 top
TP37  1.91,47.62 0 top
TP38  27.05,107.06 0 top
TP40  60.96,44.45 0 top
TP41  2.54,67.94 0 top
U1  31.75,54.61 0 top
U2  57.91,102.23 90 top
U3  31.75,71.12 270 top
U4  59.69,110.87 0 top
U5  53.72,111 0 top
U6  26.04,90.8 180 top
U$5  [UCB_CAL_350MIL]  39.37,22.48 0 top

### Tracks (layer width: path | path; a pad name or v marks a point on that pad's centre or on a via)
5V_IN  (via drill 0.2)
  Top 0.406: D1.P$2 16.34,64.94 20.32,60.96 v20.32,57.15 | v20.32,40.01 20.32,26.03 26.31,20.05 26.31,10.79 | 26.31,10.79 J16.9 | J16.8 26.31,9.87 26.31,10.79
  Bottom 0.406: v20.32,57.15 v20.32,40.01
!BUTTON_0  (via drill 0.2)
  Top 0.203: J9.4 J1.P0.28 12.7,58.42 v13.34,57.79 | S3.1 S3.2 11.6,32.98 R13.1 11.63,35.76 v12.06,36.2
  Bottom 0.203: v13.34,57.79 13.34,37.46 v12.06,36.2
!IMU_INTERRUPT  (via drill 0.2)
  Top 0.203: J1.P0.07 J11.4 | U3.12 29.28,70.12 R6.1 28.37,68.58 32.82,64.13 42.55,64.13 v43.18,64.77 | v50.8,40.01 43.18,47.62 v43.18,58.42
  Bottom 0.203: J1.P0.07 53.98,40.01 v50.8,40.01 | v43.18,58.42 v43.18,64.77
!LCD_CS
  Top 0.203: J10.8 J1.P0.18
  Bottom 0.203: J1.P0.18 53.34,68.58 50.42,65.66 A1.16
!LED_0  (via drill 0.2)
  Top 0.203: J7.5 J1.P0.25 54.1,87.12 43.3,87.12 37.64,81.47 37.64,81.46 v37.47,81.28 | D2.C 6.87,42.55 18.41,42.55 24.77,48.9 36.2,48.9 37.47,50.16 v37.47,58.42 | v37.47,64.77 v37.47,71.12
  Bottom 0.203: v37.47,58.42 v37.47,64.77 | v37.47,71.12 v37.47,81.28
!LED_1  (via drill 0.2)
  Top 0.203: J7.6 J1.P0.24 54.1,84.58 41.39,84.58 38.28,81.47 38.28,81.46 v38.1,81.28 | D3.C 8.78,41.91 19.05,41.91 25.4,48.26 36.83,48.26 38.1,49.53 v38.1,58.42 | v38.1,64.77 v38.1,71.12
  Bottom 0.203: v38.1,58.42 v38.1,64.77 | v38.1,71.12 v38.1,81.28
!LED_2  (via drill 0.2)
  Top 0.203: J7.7 J1.P0.23 54.1,82.04 39.5,82.04 v38.73,81.28 | D4.C 10.68,41.27 19.68,41.27 26.04,47.62 37.47,47.62 38.73,48.9 v38.73,58.42 | v38.73,64.77 v38.73,71.12
  Bottom 0.203: v38.73,58.42 v38.73,64.77 | v38.73,71.12 v38.73,81.28
!LIGHT_INTERRUPT  (via drill 0.2)
  Top 0.203: J1.P0.27 J7.1 | U2.4 58.56,103 59.64,101.92 59.64,99.83 58.97,99.17 v56.64,99.17 56.61,99.17 R5.1
  Bottom 0.203: v56.64,99.17 56.64,96.27 J1.P0.27
!RESET  (via drill 0.2)
  Top 0.203: J1.P0.21 J11.1 | S2.1 S2.2 12.72,111.96 R10.1 30.28,111.96 32.38,109.85 32.38,83.69 31.24,82.55 24.13,82.55 23.5,81.91 23.5,67.94 27.94,63.5 43.18,63.5 v44.45,64.77 | v44.45,58.42 44.45,52.7 48.9,48.26 v57.78,48.26
  Bottom 0.203: v44.45,64.77 v44.45,58.42 | J1.P0.21 57.78,32.38 v57.78,48.26
!SD_CS
  Top 0.203: J10.4 J1.P0.14 52.07,62.23 26.04,62.23 20.32,67.94 20.32,78.74 14.61,84.45 14.61,95.25 15.04,95.69 J17.2 17.85,95.69 19.51,94.03 R8.1
!SD_DETECT  (via drill 0.2)
  Top 0.203: J17.A 5.91,104.46 | R14.1 22.14,103.85 22.14,103.88 25.31,107.06 TP38.TESTPOINT
  Top 0.406: 5.91,104.46 v6.86,105.41
  Bottom 0.203: v6.86,105.41 8.51,107.06 TP38.TESTPOINT
+3V3  (via drill 0.2)
  Top 0.203: v62.48,112.01 60.71,113.79 59.38,113.79 59.26,113.66 C4.1 58.69,112.59 U4.1 57.82,111 57.66,111 | 57.66,111 U5.5 55.71,111 C3.1 | 57.66,111 57.66,104.9 v56.64,103.89 | R11.2 54.81,99.11 v54.61,99.31 | v52.83,99.31 52.91,99.24 R12.2
  Bottom 0.203: J15.3 59.96,21.59 v60.33,21.59 | v56.64,103.89 56.64,100.33 v56.9,100.08 | v54.61,99.31 v52.83,99.31
  pour Top: -4.45,113.66 1.27,119.38 68.58,119.38 74.93,113.03 74.93,1.9 70.48,-2.54 -4.45,-2.54 -6.99,0 -6.99,1.27 -6.99,111.12
+5V
  Top 0.406: J8.3 J1.5V D1.P$1
ANALOG_ACCEL_X
  Top 0.203: J9.3 J1.P0.29 27.74,55.88 C8.1 30.37,56.08 30.6,55.86 33.33,55.86 U1.12
ANALOG_ACCEL_Y
  Top 0.203: J9.2 J1.P0.30 27.74,53.34 C7.1 28.28,53.21 30.25,53.21 30.43,53.38 32.83,53.38 33,53.55 33,53.81 33.47,54.29 U1.10
ANALOG_ACCEL_Z
  Top 0.203: J9.1 J1.P0.31 28.37,50.8 C6.1 31.95,51 32.73,51.77 U1.8
GND  (via drill 0.2)
  Top 0.203: S2.3 S2.4 3.05,108.2 v2.79,108.2 2.55,108.45 D5.C | S3.3 S3.4 2.54,27.43 v2.54,28.58 | U5.2 51.56,110.29 51.56,109.47 52.58,108.46 | 52.58,108.46 v52.58,103.63 | U4.4 60.69,112.59 C4.2 60.58,112.7 60.58,112.14 61.47,111.25 v62.48,111.25 | U2.3 58.6,101.27 58.6,99.82 | 58.6,99.82 C10.2 59.18,100.28 v59.18,100.33 | U2.EP U2.2 57.91,100.51 58.6,99.82 | U1.7 32.08,52.14 31.8,51.87 31.11,51.87 | 30.48,51.87 31.11,51.87 | U1.6 31.43,52.18 31.11,51.87 | U1.5 30.77,52.16 30.48,51.87 | v27.43,52.07 27.63,51.87 C6.2 30.48,51.87 | C8.2 28.78,57.79 v29.21,57.79 29.84,58.42 C5.2 | U1.3 29.03,54.29 28.9,54.41 C7.2 26.98,54.41 v26.92,54.36 | C9.2 26.04,71.55 v26.04,71.37 26.04,71.32 26.77,70.59 | 26.77,70.59 C2.2 26.87,70.28 27.3,69.85 28.5,69.85 29.18,70.52 U3.11 | U3.9 27.5,71.32 26.77,70.59 | C1.2 30.68,74.93 v30.48,74.93 | U3.18 32.75,68.85 33.02,68.58 33.66,68.58 v34.29,69.22 34.29,69.85 33.62,70.52 U3.20 | C3.2 56.57,108.97 56.39,108.97 55.88,108.46 52.58,108.46
  Top 0.406: J17.MOUNT2 1.76,104.88 v2.54,105.66 | J17.MOUNT3 2.34,89.66 v3.05,89.66 | J17.B 17.56,104.39 v17.78,104.39 | J17.6 16.42,100.08 v18.54,100.08 | J17.MOUNT0 17.78,91.67 v17.78,91.44 | U6.4 24.37,89.68 v23.62,90.42 | C11.2 24.26,97.92 v24.64,98.3 | J17.MOUNT1 12.11,104.82 12.95,105.66 | 12.95,105.66 v14.22,105.66 | S2.3 12.23,106.39 12.95,105.66
  other vias: 62.99,110.49
  pour Bottom: -5.08,116.84 63.5,116.84 67.31,113.03 67.31,3.81 62.23,-1.27 0,-1.27 -7.62,6.35 -7.62,114.3
GROVE_A0  (via drill 0.2)
  Top 0.203: J9.5 J1.P0.04 12.7,60.96 v13.34,60.33 | v14.61,40.01 14.61,36.83 13.34,35.56 13.34,17.95 J12.1
  Bottom 0.203: v13.34,60.33 14.61,59.05 v14.61,40.01
GROVE_A1  (via drill 0.2)
  Top 0.203: J9.6 J1.P0.03 12.7,63.5 v13.34,62.87 | v15.88,40.01 15.88,36.2 14.61,34.92 14.61,18.69 J12.2
  Bottom 0.203: v13.34,62.87 15.88,60.33 v15.88,40.01
GROVE_D0  (via drill 0.2)
  Top 0.203: J7.3 J1.P0.02 55.12,89.66 45.09,89.66 36.83,81.41 v36.83,81.28 | v36.83,71.12 v36.83,64.77 | v36.83,58.42 36.83,50.8 35.56,49.53 v32.38,49.53 | v32.38,46.99 28.57,43.18 28.57,15.24 30.3,13.51 J13.1
  Bottom 0.203: v36.83,81.28 v36.83,71.12 | v36.83,64.77 v36.83,58.42 | v32.38,49.53 v32.38,46.99
GROVE_D1  (via drill 0.2)
  Top 0.203: J11.2 J1.P0.05 | J13.2 35.83,10.16 47.62,10.16 52.7,15.24 v52.7,16.51
  Bottom 0.203: v52.7,16.51 52.7,29.84 J1.P0.05
LCD_MISO
  Top 0.203: J10.6 J1.P0.16 50.8,68.58 50.8,70.64 A1.13
LCD_MOSI
  Top 0.203: J10.5 J1.P0.15 50.16,66.67 50.16,68.74 A1.14
LCD_SCLK
  Top 0.203: J10.7 J1.P0.17 51.44,70.48 51.44,72.55 A1.12
N$3
  Top 0.203: R4.2 24.05,109.6 18.67,109.6 17.35,110.92 15.98,110.92 14.66,109.6 D5.A
N$4
  Top 0.203: D4.A R3.2
N$5
  Top 0.203: D3.A R2.2
N$7  (via drill 0.2)
  Top 0.203: S1.1 17.78,43.82 v22.86,48.9 | v22.86,54.61 23.18,54.94 U1.2
  Bottom 0.203: v22.86,48.9 v22.86,54.61
N$18
  Top 0.406: R14.2 R9.2 22.66,97.94 C11.1 | J17.4 19.38,97.89 R7.2 21.28,97.92 C11.1 | C11.1 22.68,96.44 25.96,93.17 | 25.96,93.17 R8.2 | 25.96,93.17 26.04,93.09 U6.2 | U6.1 26.98,92.78 26.59,93.17 25.96,93.17
N$19
  Top 0.203: C2.1 28.17,70.92 U3.10
N$25
  Top 0.203: D2.A R1.2
N$50
  cutout Top: 62.23,104.14 50.8,104.14 50.8,114.3 62.23,114.3
N$51
  cutout Bottom: 62.23,104.14 50.8,104.14 50.8,114.3 62.23,114.3
SD_ENABLE  (via drill 0.2)
  Top 0.203: J7.2 J1.P0.26 55.24,92.33 38.99,92.33 v36.2,89.53 | U6.3 25.09,91.25 25.53,90.8 R15.1 29.41,89.97 29.84,89.53 v30.48,89.53
  Bottom 0.203: v30.48,89.53 v36.2,89.53
SD_MISO
  Top 0.203: J10.2 J1.P0.12 52.7,56.52 52.7,57.79 50.16,60.33 24.13,60.33 18.41,66.04 18.41,76.83 12.7,82.55 12.7,99.06 14.83,101.19 J17.7 19.4,101.19 19.81,101.6 R9.1
SD_MOSI  (via drill 0.2)
  Top 0.203: J10.1 J1.P0.11 51.44,55.25 51.44,57.15 48.9,59.69 v26.04,59.69 | R7.1 18.72,96.09 18.03,96.77 16.43,96.77 J17.3 14.88,96.79 13.97,95.88 13.97,83.82 19.68,78.1 19.68,67.31 25.4,61.59 v26.04,61.59
  Bottom 0.203: v26.04,61.59 v26.04,59.69
SD_SCLK
  Top 0.203: J10.3 J1.P0.13 53.98,57.79 50.8,60.96 24.77,60.96 19.05,66.67 19.05,77.47 13.34,83.18 13.34,98.42 13.9,98.99 J17.5
SENSORS_SCL  (via drill 0.2)
  Top 0.203: J7.10 J1.P0.19 53.98,72.64 49.53,77.09 35.81,77.09 v34.92,76.2 34.92,72.39 | U2.5 57.91,103.38 59.69,105.16 60.71,105.16 | 60.71,105.16 v60.71,107.19 60.71,109.85 U4.3 | U5.6 56.12,112 v56.13,112.01 | U3.23 34.26,71.72 34.92,72.39 | J14.1 40.64,16.05 v40.64,58.42 | v34.92,81.28 34.92,92.71 37.08,94.87 52.53,94.87 55.45,97.79 55.63,97.79 | 60.71,105.16 62.23,103.63 62.23,99.69 60.33,97.79 55.63,97.79 | 34.92,72.39 39.37,72.39 40.64,71.12 v40.64,64.77 | R11.1 55.68,97.84 55.63,97.79
  Bottom 0.203: v40.64,58.42 v40.64,64.77 | v34.92,81.28 v34.92,76.2 | v56.13,112.01 57.66,110.49 57.66,107.7 58.17,107.19 v60.71,107.19
SENSORS_SDA  (via drill 0.2)
  Top 0.203: J7.9 J1.P0.20 51.44,79.63 34.54,79.63 33.66,78.74 | U4.2 58.67,109.85 58.67,108.2 | U5.1 53.3,113.03 v56.13,113.03 | 58.67,108.2 58.67,105.08 57.26,103.67 U2.6 56.04,103.16 53.77,100.89 R12.1 53.77,97.84 53.34,97.41 36.45,97.41 33.66,94.61 33.66,78.74 | U3.24 33.66,72.52 v33.66,73.66 33.66,78.74 | J14.2 41.91,16.78 v41.91,58.42 | v36.2,73.66 40.64,73.66 41.91,72.39 v41.91,64.77 | v59.18,108.2 58.67,108.2
  Bottom 0.203: v41.91,58.42 v41.91,64.77 | v36.2,73.66 v33.66,73.66 | v56.13,113.03 59.18,109.98 v59.18,108.2
SWITCH_0  (via drill 0.2)
  Top 0.203: J7.8 J1.P0.22 | S4.IN 11.43,20.32 v11.43,22.23 | v16.51,22.23 19.05,24.77 19.05,38.73 v17.78,40.01 | v22.23,67.94 22.23,83.18 23.62,84.58 v30.48,84.58
  Bottom 0.203: v11.43,22.23 v16.51,22.23 | v17.78,40.01 17.78,63.5 v22.23,67.94 | J1.P0.22 49.02,84.58 37.34,84.58 v30.48,84.58
UART_RX
  Top 0.203: J11.5 J1.P0.08 49.53,34.29 49.53,21.86 J15.2 49.01,8.64 47.15,8.64 J16.2
UART_TX
  Top 0.203: J11.3 J1.P0.06 50.93,30.61 50.93,22.73 52.2,21.46 56.01,21.46 57.78,19.69 57.78,15.41 J15.1 49.48,7.11 J16.1

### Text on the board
tPlace: RESET | POWER | MS5637 / PRESS | SI7021 / TEMP & / HUMID | MAX44009 / LIGHT | !LIGHT_INT | SD_EN | GROVE_D0 | SD Card | !LED_0 | !LED_1 | !LED_2 | SWITCH_0 | MPU-9250 / I2C ACCELEROMETER / GYRO & MAGNETOMETER | SDA | +Y | SCL | +Z | . | !LCD_CS | LCD_SCLK | GND | +X | LCD_MISO | GROVE_A1 | LCD_MOSI | GROVE_A0 | ADXL327 / ANALOG ACCELEROMETER | !SD_CS | !BUTTON_0 | ACCEL_X | SD_SCLK | +Y | SD_MISO | ACCEL_Y | +Z | . | ACCEL_Z | SD_MOSI | ACCEL / SELF TEST | +X | GND | GND | 0 | 1 | 2 | !IMU_INT | GROVE_D1 | Berkeley Buckler | C | B. Ghena, N. Jackson | BUTTON_0 | July 2020 | GND | GND | GND | GND | VCC | VCC | VCC | VCC | A1 | D1 | SDA | RX | A0 | D0 | SCL | TX | SWITCH_0 | GND | GND
tNames: SD_DETECT | J2 | J1 | J4 | J3 | J5 | LO | HI

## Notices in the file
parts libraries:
SparkFun-Aesthetics: Licensing: Creative Commons ShareAlike 4.0 International - https://creativecommons.org/licenses/by-sa/4.0
SparkFun-Connectors: Licensing: CC v3.0 Share-Alike You are welcome to use this library for commercial purposes.
